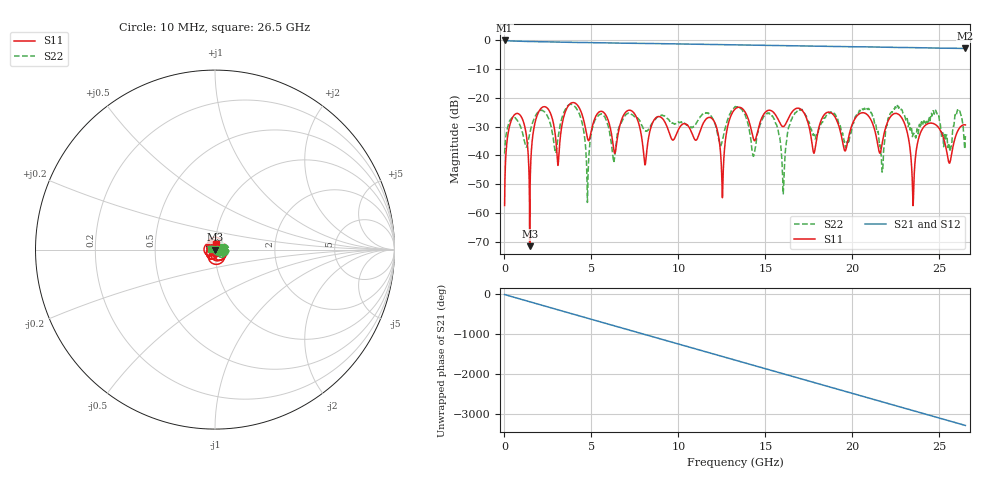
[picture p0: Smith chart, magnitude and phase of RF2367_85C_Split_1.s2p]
!Keysight Technologies,N5245B,MY55451909,A.13.80.08
!Automatic Fixture Removal (AFR)
!Date: Thursday, August 27, 2020, 03:56:27
!S2P File: Measurements: S11,S21,S12,S22:
# MHz S  RI  R 50
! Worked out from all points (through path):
!   2650 points, 10 MHz to 26.5 GHz, reference 50 ohm
!   highest |S21| = -0.01 dB at 10 MHz (marker M1); lowest = -2.8 dB at 26.48 GHz (marker M2)
!   group delay of S21, straight-line fit = 344 ps
!   lowest |S11| = -71.5 dB at 1.45 GHz (marker M3), VSWR 1.00, Z = 50 - j0.0264 ohm
!   |S11| at or under -10 dB: start of sweep to end of sweep
!   |S22| runs from -56.3 to -22.2 dB; largest |S21 - S12| = 1.4e-15
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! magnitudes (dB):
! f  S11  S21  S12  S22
! 10 MHz  -57.4  0.0  0.0  -39.3
! 640 MHz  -25.5  -0.2  -0.2  -27.0
! 1.45 GHz  -71.5  -0.4  -0.4  -32.4
! 2.11 GHz  -23.6  -0.5  -0.5  -24.3
! 3.07 GHz  -43.4  -0.6  -0.6  -34.3
! 4.43 GHz  -25.2  -0.7  -0.7  -27.8
! 4.78 GHz  -34.2  -0.7  -0.7  -54.4
! 5.46 GHz  -24.8  -0.8  -0.8  -25.9
! 8.09 GHz  -43.3  -1.0  -1.0  -31.3
! 8.84 GHz  -26.5  -1.1  -1.1  -26.5
! 11.91 GHz  -27.0  -1.4  -1.4  -26.6
! 12.53 GHz  -54.7  -1.4  -1.4  -34.8
! 13.26 GHz  -23.8  -1.5  -1.5  -23.0
! 15.4 GHz  -24.7  -1.7  -1.7  -26.3
! 16.03 GHz  -30.0  -1.8  -1.8  -53.3
! 16.68 GHz  -24.0  -1.8  -1.8  -25.4
! 17.67 GHz  -35.3  -1.9  -1.9  -31.6
! 22.09 GHz  -27.6  -2.4  -2.4  -27.0
! 23.5 GHz  -57.1  -2.5  -2.5  -32.5
! 24.17 GHz  -29.7  -2.6  -2.6  -29.1
! 26.48 GHz  -29.4  -2.8  -2.8  -36.1
! 26.5 GHz  -29.4  -2.8  -2.8  -33.3
